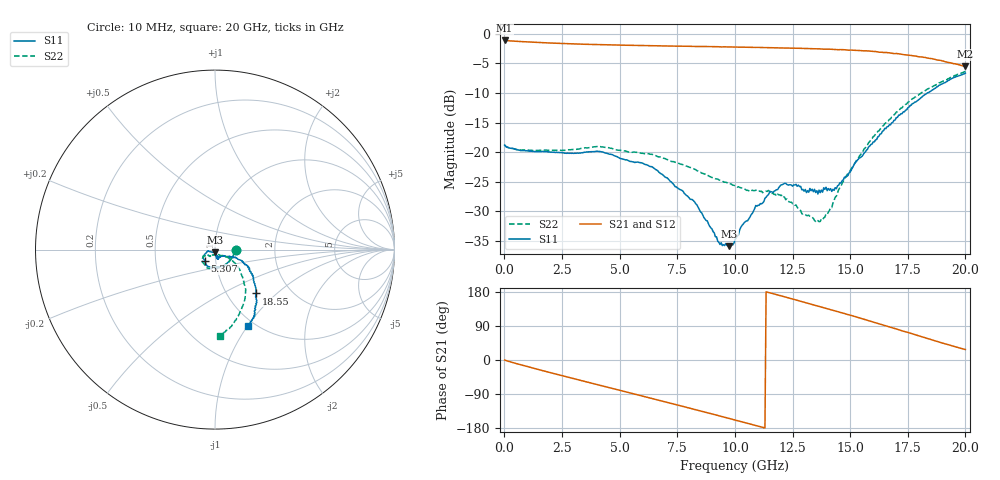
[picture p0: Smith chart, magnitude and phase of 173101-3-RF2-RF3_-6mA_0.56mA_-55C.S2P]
!  2-Port S-parameters saved by WinCal
! VAR MeasName=S-Parameters (CALIBRATED_DATA) read from VNA (N5242A)
! VAR MeasDate=2017-7-20 10:23:39
! VAR NAME=173101-3-RF2-RF3_-6mA_0.56mA_-55C
! VAR FILENAME=173101-3-RF2-RF3_-6mA_0.56mA_-55C.S2P
! VAR DATE=2017-7-20 10:23:40
! VAR PHYS_PORTS=1,2
# Hz S DB R 50
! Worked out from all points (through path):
!   401 points, 10 MHz to 20 GHz, reference 50 ohm
!   highest |S21| = -1.10 dB at 10 MHz (marker M1); lowest = -5.5 dB at 20 GHz (marker M2)
!   group delay of S21, straight-line fit = 45.6 ps
!   lowest |S11| = -35.9 dB at 9.755 GHz (marker M3), VSWR 1.03, Z = 50 - j1.6 ohm
!   |S11| at or under -10 dB: start of sweep to 18.35 GHz
!   |S22| runs from -31.8 to -6.4 dB; largest |S21 - S12| = 0.0094
!   S11 on the Smith chart (normalised r, x): 10 MHz: 1.26, -0.01; 5.307 GHz: 0.88, -0.11; 18.55 GHz: 1.36, -0.75; 20 GHz: 0.92, -1.01
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1e7  -18.81 -2.4  -1.10 -0.1  -1.11 -0.1  -18.78 -2.4
1.559225e9  -19.92 -55.9  -1.46 -26.5  -1.47 -26.5  -19.70 -55.8
3.358325e9  -20.11 -99.6  -1.73 -54.6  -1.74 -54.7  -19.36 -97.2
4.157925e9  -19.91 -115.4  -1.82 -66.9  -1.83 -66.9  -19.07 -112.3
5.30735e9  -21.31 -132.1  -1.91 -84.6  -1.94 -84.6  -19.89 -125.7
6.70665e9  -23.40 -152.8  -2.01 -106.4  -2.01 -106.3  -20.82 -142.0
8.255875e9  -28.46 -165.6  -2.12 -130.5  -2.14 -130.5  -22.91 -151.2
9.355325e9  -35.65 -117.8  -2.19 -148.0  -2.18 -148.0  -24.77 -144.8
9.755125e9  -35.93 -87.6  -2.20 -154.4  -2.21 -154.5  -25.35 -145.1
1.0005e10  -34.86 -84.2  -2.22 -158.3  -2.24 -158.4  -25.73 -144.3
1.030485e10  -32.44 -77.3  -2.23 -163.1  -2.25 -163.2  -26.07 -139.5
1.090455e10  -29.05 -74.5  -2.28 -172.7  -2.30 -172.8  -26.47 -131.1
1.205398e10  -25.52 -76.2  -2.37 168.5  -2.39 168.5  -27.20 -124.4
1.335332e10  -26.28 -66.9  -2.50 146.7  -2.47 146.6  -31.02 -93.0
1.375312e10  -26.43 -62.8  -2.55 139.8  -2.55 139.7  -31.31 -80.9
1.430285e10  -26.46 -50.4  -2.63 130.4  -2.65 130.4  -28.20 -51.2
1.475262e10  -24.25 -35.8  -2.68 122.5  -2.69 122.4  -24.55 -36.0
1.535232e10  -21.19 -25.2  -2.80 112.1  -2.80 111.7  -21.03 -31.4
1.670165e10  -15.37 -23.4  -3.19 87.3  -3.27 86.9  -14.48 -41.2
1.76012e10  -12.14 -33.1  -3.63 70.9  -3.64 70.8  -11.26 -51.5
1.855072e10  -9.51 -46.9  -4.18 53.0  -4.28 53.1  -8.97 -65.0
2e10  -6.62 -66.6  -5.49 27.7  -5.55 28.3  -6.36 -86.7
